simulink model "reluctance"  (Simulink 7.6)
settings: Solver=ode15s  StartTime=0.0  StopTime=0.02  RelTol=1e-3
StopFcn:
  | close all
  | 
  | load VI_partie_electrique.mat
  | plotyy(x(1,:),x(2,:),x(1,:),x(3,:))
  | grid
  | title('Tension et courant dans le coté électrique du convertisseur')
  | 
  | figure
  | load MMF_et_flux.mat
  | plotyy(y(1,:),y(2,:),y(1,:),y(3,:))
  | grid
  | title('Flux magnétique et MMF')
libraries: fl_lib x10, nesl_utility x6

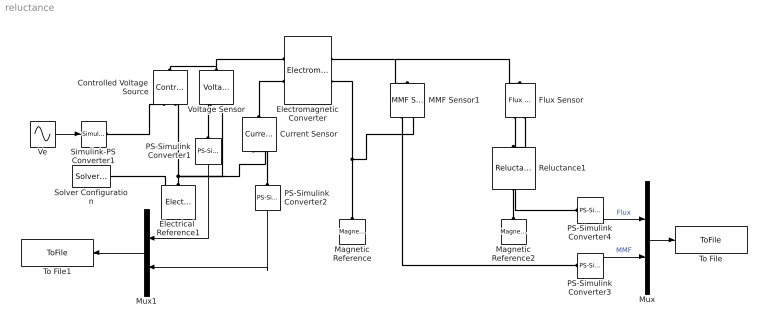
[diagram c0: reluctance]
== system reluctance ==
  Controlled Voltage Source : fl_lib/Electrical/Electrical Sources/Controlled Voltage Source  DialogController=NetworkEngine.DynNeDlgSource  SystemSampleTime=-1  i_Log=off  v_Log=off  LocalVarNames=|i|v  LocalVarDescs=|i|v  LocalVarLogging=[0 0]
  Current Sensor : fl_lib/Electrical/Electrical Sensors/Current Sensor  DialogController=NetworkEngine.DynNeDlgSource  SystemSampleTime=-1  i1_Log=off  v1_Log=off  LocalVarNames=|i1|v1  LocalVarDescs=|i1|v1  LocalVarLogging=[0 0]
  Electrical  Reference1 : fl_lib/Electrical/Electrical Elements/Electrical Reference  DialogController=NetworkEngine.DynNeDlgSource  SystemSampleTime=-1  i_Log=off  LocalVarNames=|i  LocalVarDescs=|i  LocalVarLogging=0
  Electromagnetic Converter : fl_lib/Magnetic/Magnetic Elements/Electromagnetic Converter  DialogController=NetworkEngine.DynNeDlgSource  SystemSampleTime=-1  Nw=2000  i_Log=off  v_Log=off  mmf_Log=off  phi_Log=off  LocalVarNames=|i|v|mmf|phi  LocalVarDescs=|i|v|mmf|phi  LocalVarLogging=[0 0 0 0]
  Flux Sensor : fl_lib/Magnetic/Magnetic Sensors/Flux Sensor  DialogController=NetworkEngine.DynNeDlgSource  SystemSampleTime=-1  phi_Log=off  mmf_Log=off  LocalVarNames=|phi|mmf  LocalVarDescs=|phi|mmf  LocalVarLogging=[0 0]
  MMF Sensor1 : fl_lib/Magnetic/Magnetic Sensors/MMF Sensor  DialogController=NetworkEngine.DynNeDlgSource  SystemSampleTime=-1  phi_Log=off  mmf_Log=off  LocalVarNames=|phi|mmf  LocalVarDescs=|phi|mmf  LocalVarLogging=[0 0]
  Magnetic Reference : fl_lib/Magnetic/Magnetic Elements/Magnetic Reference  DialogController=NetworkEngine.DynNeDlgSource  SystemSampleTime=-1  phi_Log=off  LocalVarNames=|phi  LocalVarDescs=|phi  LocalVarLogging=0
  Magnetic Reference2 : fl_lib/Magnetic/Magnetic Elements/Magnetic Reference  DialogController=NetworkEngine.DynNeDlgSource  SystemSampleTime=-1  phi_Log=off  LocalVarNames=|phi  LocalVarDescs=|phi  LocalVarLogging=0
  Mux : Mux  Inputs=2
  Mux1 : Mux  Inputs=2
  PS-Simulink Converter{1..4} (4 alike) : nesl_utility/PS-Simulink Converter  DialogController=NetworkEngine.DynNeUtilDlgSource  SystemSampleTime=-1  PhysicalDomain=network_engine_domain  LeftPortType=input  RightPortType=output  SubClassName=ps_output  Unit=1  AffineConversion=off
  Reluctance1 : fl_lib/Magnetic/Magnetic Elements/Reluctance  DialogController=NetworkEngine.DynNeDlgSource  SystemSampleTime=-1  g=0.001 m  CSA=0.01 m^2  mur=1  phi_Log=off  mmf_Log=off  LocalVarNames=|phi|mmf  LocalVarDescs=|phi|mmf  LocalVarLogging=[0 0]
  Simulink-PS Converter1 : nesl_utility/Simulink-PS Converter  DialogController=NetworkEngine.DynNeUtilDlgSource  SystemSampleTime=-1  PhysicalDomain=network_engine_domain  LeftPortType=input  RightPortType=output  SubClassName=ps_input  Unit=1  AffineConversion=off  InputFilterTimeConstant=.001  UdotUserProvided=0
  Solver Configuration : nesl_utility/Solver Configuration  DialogController=NetworkEngine.DynNeUtilDlgSource  SystemSampleTime=-1  PhysicalDomain=network_engine_domain  LeftPortType=input  RightPortType=generic  SubClassName=solver  Accelerate=off  Profile=off  ResidualTolerance=1e-9  MaxNonlinIter=3  MaxModeIter=2  DoFixedCost=off  UseLocalSampling=off  DoDC=off  LinearAlgebra=Sparse  LocalSolverSampleTime=.001  LocalSolverChoice=NE_BACKWARD_EULER_ADVANCER  UseLocalSolver=off
  To File : ToFile  Filename=MMF_et_flux  MatrixName=y
  To File1 : ToFile  Filename=VI_partie_electrique  MatrixName=x
  Ve : Sin  Amplitude=120  Frequency=4*pi*60  Phase=pi/2  SampleTime=0
  Voltage Sensor : fl_lib/Electrical/Electrical Sensors/Voltage Sensor  DialogController=NetworkEngine.DynNeDlgSource  SystemSampleTime=-1  i1_Log=off  v1_Log=off  LocalVarNames=|i1|v1  LocalVarDescs=|i1|v1  LocalVarLogging=[0 0]
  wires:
  Ve/1 -> Simulink-PS Converter1/1
  Mux/1 -> To File/1
  PS-Simulink Converter4/1 -> Mux/1  "Flux"
  PS-Simulink Converter3/1 -> Mux/2  "MMF"
  PS-Simulink Converter1/1 -> Mux1/1
  PS-Simulink Converter2/1 -> Mux1/2
  Mux1/1 -> To File1/1
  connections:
  Electromagnetic Converter/RConn1 -- MMF Sensor1/LConn1 -- Flux Sensor/LConn1
  Magnetic Reference/LConn1 -- Electromagnetic Converter/RConn2 -- MMF Sensor1/RConn2
  Simulink-PS Converter1/RConn1 -- Controlled Voltage Source/RConn1
  Controlled Voltage Source/LConn1 -- Electromagnetic Converter/LConn1 -- Voltage Sensor/LConn1
  Electrical  Reference1/LConn1 -- Voltage Sensor/RConn2 -- Current Sensor/RConn2 -- Controlled Voltage Source/RConn2 -- Solver Configuration/RConn1
  MMF Sensor1/RConn1 -- PS-Simulink Converter3/LConn1
  Current Sensor/LConn1 -- Electromagnetic Converter/LConn2
  PS-Simulink Converter1/LConn1 -- Voltage Sensor/RConn1
  PS-Simulink Converter2/LConn1 -- Current Sensor/RConn1
  Reluctance1/RConn1 -- Magnetic Reference2/LConn1
  Flux Sensor/RConn2 -- Reluctance1/LConn1
  Flux Sensor/RConn1 -- PS-Simulink Converter4/LConn1
